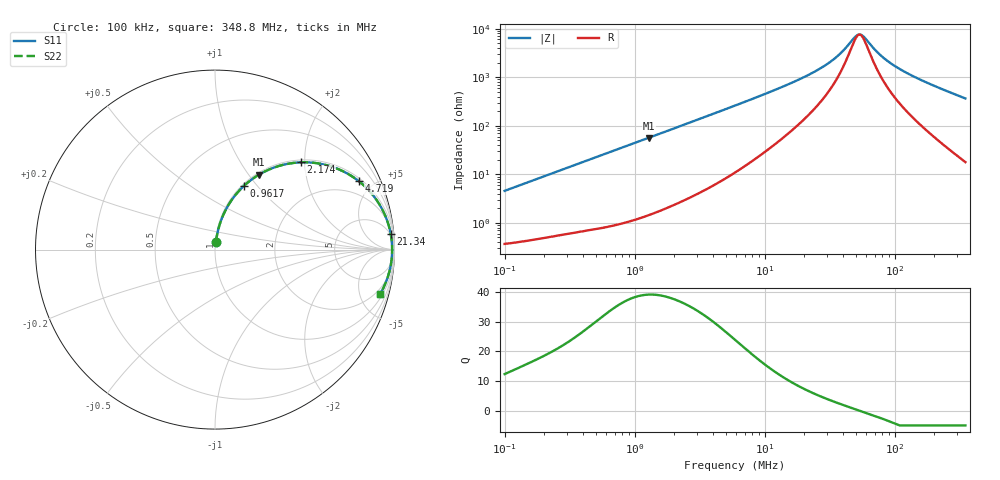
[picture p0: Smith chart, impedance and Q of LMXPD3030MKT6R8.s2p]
! LMXPD3030MKT6R8  S-PARAMETER MODEL  ( General Type )
! Model Generated by TAIYO YUDEN Corporation (http://www.ty-top.com)
! Version 1.0
! TAIYO YUDEN Control No. 191023NI43SB-FBB
! Copyright(c) 2019 TAIYO YUDEN CO.,LTD. All Rights Reserved.
! Product Description (link to TY-COMPAS)
! https://ds.yuden.co.jp/TYCOMPAS/or/detail?pn=LMXPD3030MKT6R8M&u=M
! Products Name : Inductors
! Characteristics :
!  Inductance : 6.8 uH , SRF(min) : 40 MHz , DC Resistance(max) : 0.36 Ohm
!  Rated Current : Saturation :950 mA , Temp Rise : 650 mA
!  Case Size : 3.0 x 3.0 / 0.118 x 0.118 [mm/inch] , Thickness : 1.2 / 0.047 [mm/inch]
!  (Conditions: Temperature = 25 degC , DC Bias Current/Voltage = 0A / 0V)
! External Node Assignments :
!  1  o---GGG---o  2
! GND o---------o GND
! Frequency Range : 0.1MHz  -  348.750116MHz  [ 402 STEP ]
# MHz S RI R 50
! Freq[MHz].  S11 Real  S11 Imag  S21 Real  S21 Imag  S12 Real  S12 Imag  S22 Real  S22 Imag
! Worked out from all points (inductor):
!   401 points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, 100 kHz to 348.8 MHz, reference 50 ohm
!   read as one part in series: L = 7.21 uH near 104.2 kHz
!   highest Q = 39.2 at 1.279 MHz (marker M1), where L = 7 uH
!   self-resonance near 53.51 MHz
!   S11 on the Smith chart (normalised r, x): 100 kHz: 1.01, +0.09; 961.7 kHz: 1.02, +0.85; 2.174 MHz: 1.05, +1.91; 4.719 MHz: 1.15, +4.14; 21.34 MHz: 4, +22; 348.8 MHz: 1.36, -7.29
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0.1  0.00571 0.045  0.9943 -0.045  0.9943 -0.045  0.00571 0.045
0.392077  0.0355 0.167  0.9645 -0.167  0.9645 -0.167  0.0355 0.167
0.63962  0.0806 0.2578  0.9194 -0.2578  0.9194 -0.2578  0.0806 0.2578
0.961718  0.1588 0.3526  0.8412 -0.3526  0.8412 -0.3526  0.1588 0.3526
1.279487  0.2462 0.4182  0.7538 -0.4182  0.7538 -0.4182  0.2462 0.4182
1.537242  0.3177 0.4529  0.6823 -0.4529  0.6823 -0.4529  0.3177 0.4529
2.174198  0.4768 0.4861  0.5232 -0.4861  0.5232 -0.4861  0.4768 0.4861
3.075077  0.6406 0.4652  0.3594 -0.4652  0.3594 -0.4652  0.6406 0.4652
4.71887  0.8022 0.3806  0.1978 -0.3806  0.1978 -0.3806  0.8022 0.3806
5.905507  0.861 0.3257  0.139 -0.3257  0.139 -0.3257  0.861 0.3257
10.03508  0.9412 0.2053  0.0588 -0.2053  0.0588 -0.2053  0.9412 0.2053
21.34043  0.9789 0.0876  0.0211 -0.0876  0.0211 -0.0876  0.9789 0.0876
23.15412  0.9806 0.0782  0.0194 -0.0782  0.0194 -0.0782  0.9806 0.0782
34.11126  0.9854 0.039  0.0146 -0.039  0.0146 -0.039  0.9854 0.039
40.15578  0.9864 0.0244  0.0136 -0.0244  0.0136 -0.0244  0.9864 0.0244
49.23919  0.9869 0.00697  0.0131 -0.00697  0.0131 -0.00697  0.9869 0.00697
53.42396  0.987 0.000127  0.013 -0.000127  0.013 -0.000127  0.987 0.000127
57.96438  0.9869 -0.00672  0.0131 0.00672  0.0131 0.00672  0.9869 -0.00672
74.03492  0.9862 -0.0277  0.0138 0.0277  0.0138 0.0277  0.9862 -0.0277
90.78195  0.9848 -0.0463  0.0152 0.0463  0.0152 0.0463  0.9848 -0.0463
154.2634  0.9757 -0.1051  0.0243 0.1051  0.0243 0.1051  0.9757 -0.1051
348.7501  0.9196 -0.2485  0.0804 0.2485  0.0804 0.2485  0.9196 -0.2485
